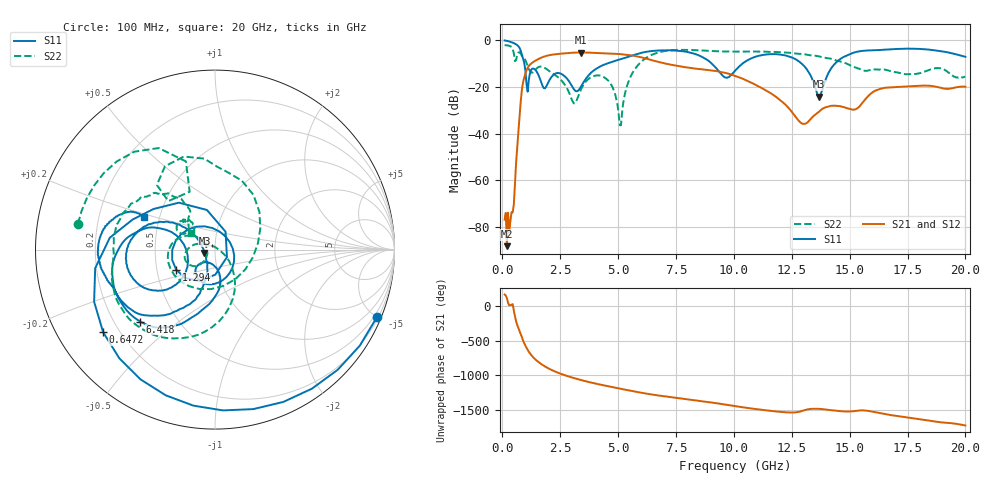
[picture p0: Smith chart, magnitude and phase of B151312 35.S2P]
!  2-Port S-parameters saved by WinCal
! VAR MeasName=S-Parameters (CALIBRATED_DATA) read from VNA (N5244A)
! VAR MeasDate=12/8/2015 5:46:22 PM
! VAR NAME=B151312 35
! VAR FILENAME=B151312 35.S2P
! VAR DATE=12/8/2015 5:46:22 PM
! VAR PHYS_PORTS=1,2
# Hz S DB R 50
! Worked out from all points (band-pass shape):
!   401 points, 100 MHz to 20 GHz, reference 50 ohm
!   highest |S21| = -5.35 dB at 3.384 GHz (marker M1); lowest = -88.1 dB at 199.5 MHz (marker M2)
!   |S21| within 3 dB of the highest: 1.518 GHz to 6.359 GHz (4.841 GHz wide, 123 % of centre)
!   lowest |S11| = -24.2 dB at 13.68 GHz (marker M3), VSWR 1.13, Z = 44.4 - j1.71 ohm
!   |S11| at or under -10 dB: 951.3 MHz to 4.547 GHz (3.596 GHz wide, 131 % of centre); 9.037 GHz to 10.38 GHz (1.347 GHz wide, 13.9 % of centre); 12.92 GHz to 14.38 GHz (1.464 GHz wide, 10.7 % of centre)
!   |S22| runs from -36.4 to -2.2 dB; largest |S21 - S12| = 0.0022
!   S11 on the Smith chart (normalised r, x): 100 MHz: 0.29, -4.99; 647.2 MHz: 0.14, -0.32; 1.294 GHz: 0.63, -0.15; 6.418 GHz: 0.31, -0.37; 20 GHz: 0.41, +0.18
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1e8  -0.20 -22.6  -76.79 161.0  -81.95 160.6  -2.19 169.3
1.995e8  -0.38 -44.4  -88.12 108.2  -95.40 124.2  -2.28 158.2
3.985e8  -0.94 -87.2  -73.63 13.1  -74.04 -21.8  -3.01 129.5
6.4725e8  -2.22 -143.5  -45.44 81.9  -45.33 82.1  -6.30 132.0
8.96e8  -7.73 146.6  -18.14 -138.6  -18.14 -138.6  -7.22 80.3
1.294e9  -12.26 -152.3  -9.71 -6.5  -9.71 -6.6  -13.98 -55.4
2.04025e9  -17.08 -46.0  -6.48 171.1  -6.47 171.1  -13.37 163.1
2.63725e9  -15.05 -126.5  -5.74 88.5  -5.74 88.5  -18.31 145.1
3.3835e9  -20.19 -87.8  -5.35 13.2  -5.34 13.2  -21.50 -134.0
3.43325e9  -19.34 -84.1  -5.35 8.8  -5.35 8.8  -20.40 -134.1
4.42825e9  -10.43 -95.5  -5.69 -67.7  -5.69 -67.7  -16.19 -178.9
5.12475e9  -8.17 -107.8  -6.06 -114.7  -6.04 -114.6  -36.45 18.0
5.5725e9  -6.73 -115.3  -6.56 -143.9  -6.55 -143.9  -15.04 -53.1
6.41825e9  -4.76 -136.1  -8.52 165.9  -8.49 165.8  -6.50 -99.4
6.7665e9  -4.48 -145.1  -9.42 149.0  -9.42 148.9  -5.27 -114.7
1.005e10  -13.17 -140.8  -15.30 -3.4  -15.29 -3.2  -4.94 179.9
1.199025e10  -6.18 179.6  -25.58 -85.0  -25.56 -85.3  -5.22 157.6
1.338325e10  -16.60 145.0  -33.13 -41.4  -33.08 -41.8  -6.64 138.3
1.368175e10  -24.20 -161.9  -30.62 -42.3  -30.58 -42.1  -7.02 135.7
1.4627e10  -7.90 -121.9  -28.38 -76.4  -28.34 -76.7  -9.28 123.9
1.67165e10  -4.04 -166.5  -20.30 -128.6  -20.21 -129.4  -13.15 136.1
2e10  -7.17 155.3  -20.01 78.9  -20.05 78.6  -15.73 144.8
